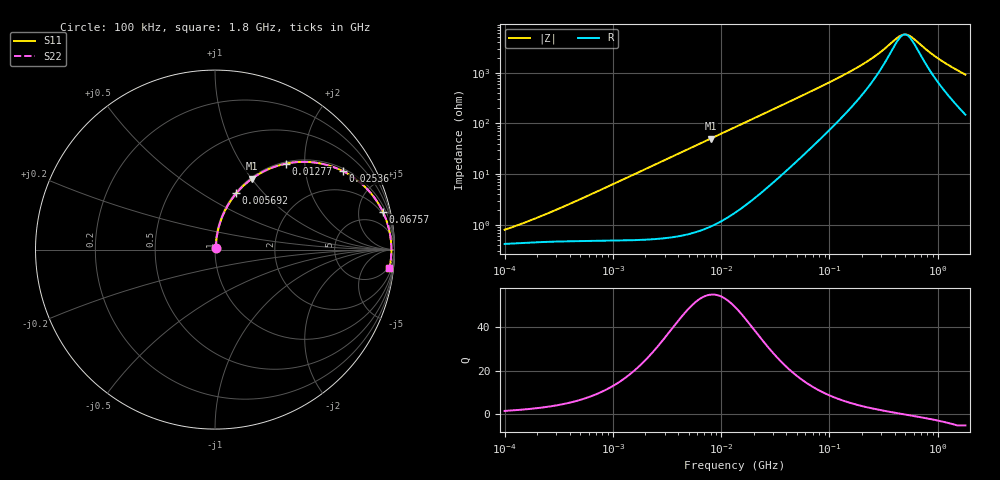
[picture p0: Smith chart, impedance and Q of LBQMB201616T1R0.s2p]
! LBQMB201616T1R0  S-PARAMETER MODEL  ( General Type )
! Model Generated by TAIYO YUDEN Corporation (http://www.ty-top.com)
! Version 1.0
! TAIYO YUDEN Control No. 191025NI43SB-FBB
! Copyright(c) 2019 TAIYO YUDEN CO.,LTD. All Rights Reserved.
! Product Description (link to TY-COMPAS)
! https://ds.yuden.co.jp/TYCOMPAS/or/detail?pn=LBQMB201616T1R0J&u=M
! Products Name : Inductors
! Characteristics :
!  Inductance : 1.0 uH , SRF(min) : 220 MHz , DC Resistance(max) : 0.494 Ohm , Rated Current : 385 mA
!  Case Size : 2.0 x 1.6 / 0.079 x 0.063 [mm/inch] , Thickness : 1.6 / 0.063 [mm/inch]
!  (Conditions: Temperature = 25 degC , DC Bias Current/Voltage = 0A / 0V)
! External Node Assignments :
!  1  o---GGG---o  2
! GND o---------o GND
! Frequency Range : 0.1MHz  -  1800MHz  [ 402 STEP ]
# MHz S RI R 50
! Freq[MHz].  S11 Real  S11 Imag  S21 Real  S21 Imag  S12 Real  S12 Imag  S22 Real  S22 Imag
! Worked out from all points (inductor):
!   401 points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, 100 kHz to 1.8 GHz, reference 50 ohm
!   read as one part in series: L = 1.02 uH near 213.7 kHz
!   highest Q = 54.5 at 8.021 MHz (marker M1), where L = 1 uH
!   self-resonance near 497.5 MHz
!   S11 on the Smith chart (normalised r, x): 100 kHz: 1.01, +0.01; 5.692 MHz: 1.01, +0.72; 12.77 MHz: 1.03, +1.61; 25.36 MHz: 1.10, +3.19; 67.57 MHz: 1.66, +8.60; 1.8 GHz: 4, -18
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0.1  0.00421 0.00671  0.9958 -0.00671  0.9958 -0.00671  0.00421 0.00671
0.203473  0.00467 0.0131  0.9953 -0.0131  0.9953 -0.0131  0.00467 0.0131
0.516129  0.00579 0.0323  0.9942 -0.0323  0.9942 -0.0323  0.00579 0.0323
1.277529  0.0112 0.0791  0.9888 -0.0791  0.9888 -0.0791  0.0112 0.0791
2.66389  0.0321 0.1612  0.9679 -0.1612  0.9679 -0.1612  0.0321 0.1612
5.692459  0.1182 0.3132  0.8818 -0.3132  0.8818 -0.3132  0.1182 0.3132
8.02111  0.207 0.3961  0.793 -0.3961  0.793 -0.3961  0.207 0.3961
12.77497  0.3942 0.4788  0.6058 -0.4788  0.6058 -0.4788  0.3942 0.4788
13.41641  0.4174 0.483  0.5826 -0.483  0.5826 -0.483  0.4174 0.483
18.00091  0.5604 0.4845  0.4396 -0.4845  0.4396 -0.4845  0.5604 0.4845
25.36465  0.7125 0.4374  0.2875 -0.4374  0.2875 -0.4374  0.7125 0.4374
40.39749  0.8557 0.3289  0.1443 -0.3289  0.1443 -0.3289  0.8557 0.3289
67.57036  0.9344 0.2122  0.0656 -0.2122  0.0656 -0.2122  0.9344 0.2122
69.24595  0.9367 0.2074  0.0633 -0.2074  0.0633 -0.2074  0.9367 0.2074
189.0427  0.9779 0.0692  0.0221 -0.0692  0.0221 -0.0692  0.9779 0.0692
266.3756  0.9811 0.0411  0.0189 -0.0411  0.0189 -0.0411  0.9811 0.0411
357.3983  0.9824 0.0208  0.0176 -0.0208  0.0176 -0.0208  0.9824 0.0208
456.5984  0.9828 0.00531  0.0172 -0.00531  0.0172 -0.00531  0.9828 0.00531
528.8877  0.9828 -0.00378  0.0172 0.00378  0.0172 0.00378  0.9828 -0.00378
583.3325  0.9827 -0.00988  0.0173 0.00988  0.0173 0.00988  0.9827 -0.00988
1024.694  0.9804 -0.0485  0.0196 0.0485  0.0196 0.0485  0.9804 -0.0485
1800  0.9721 -0.1021  0.0279 0.1021  0.0279 0.1021  0.9721 -0.1021
